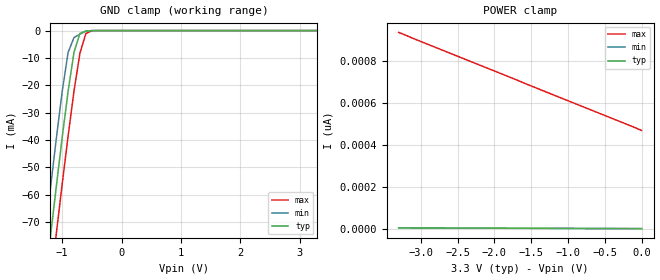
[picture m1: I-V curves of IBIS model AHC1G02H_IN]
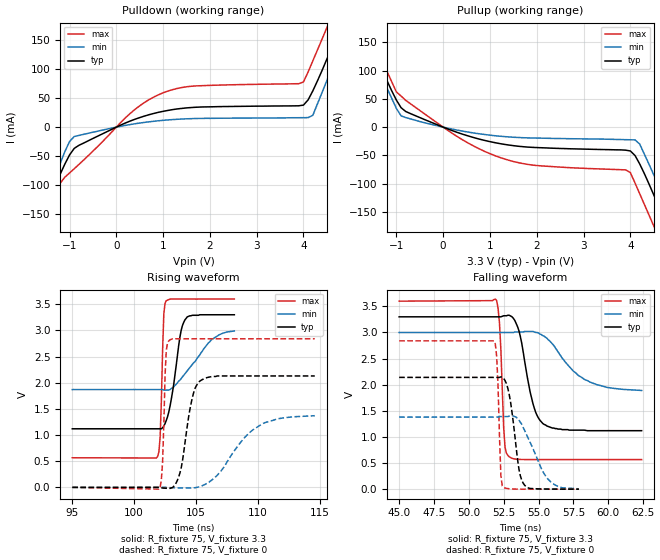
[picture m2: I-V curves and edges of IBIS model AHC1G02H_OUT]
| TEXAS INSTRUMENTS INCORPORATED
| Standard Linear and Logic Group
| IBIS Model of SN74AHC1G02H
| SINGLE 2-INPUT POSITIVE-NOR GATE
| CMPAK-5 5-pin (DCK) Package
[IBIS Ver]   2.1
[Comment Char]  |_char
[File name]   ul02_3c.ibs
[File Rev]   2.0
[Date]   May 11, 2000
[Source]   Data created from SPICE simulations at Hitachi,Ltd.
[Notes]   The following is an IBIS List for the AHC1G02H.
|   Please contact sllibis@ti.com with questions and
|   comments concerning SLL IBIS models.
[Disclaimer] Property of Texas Instruments Incorporated.  Unauthorized
   reproduction and/or distribution is strictly prohibited.
   This product is protected under copyright law.
   Created 2000, (C) Copyright 2000, Texas Instruments Inc.,
   All Rights Reserved.
   UNLESS THERE IS A SIGNED, WRITTEN AGREEMENT TO THE
   CONTRARY, TEXAS INSTRUMENTS () IS PROVIDING THE IBIS
   MODELS  AND WITHOUT ANY WARRANTY, EXPRESSED OR
   IMPLIED.  TI assumes no liability for:
   1) the accuracy of the IBIS models provided to your
   company;
   2) the proper functioning of these IBIS Models in your
   design or for any resulting applications; or
   3) infringement of patents, copyrights or intellectual
   property rights resulting from your use of these IBIS
   models.
   TI provides IBIS Models as a service to our customers.
   You and your company shall not distribute, sell or give
   these models to anyone else without prior written
   permission from TI.
   TI reserves the right to make changes to our products or
   to discontinue any semiconductor product or service
   without notice, and advises our customers to obtain the
   latest version of relevant information to verify, before
   placing orders, that the information being relied on is
   current.
   Please be aware that your receipt and use of the IBIS
   information provided shall serve as acceptance of these
   terms and conditions.  If you do not accept these terms,
   you should return or destroy the IBIS models and any
   other accompanying information immediately.
|   Component AHC1G02H
[Component]   AHC1G02H
[Manufacturer]   Hitachi, Ltd.
[Package]
|   typ   min   max
R_pkg   0.090   0.051   0.105
L_pkg   1.500nH   0.940nH   1.700nH
C_pkg   0.170pF   0.110pF   0.360pF
[Pin]   signal_name   model_name   R_pin   L_pin   C_pin
1   A   AHC1G02H_IN   0.098   1.590nH   0.110pF
2   B   AHC1G02H_IN   0.051   0.940nH   0.170pF
3   GND   GND   0.092   1.590nH   0.360pF
4   Y   AHC1G02H_OUT   0.105   1.700nH   0.110pF
5   VCC   POWER   0.104   1.690nH   0.110pF
| Models and submodels in the file (2): AHC1G02H_IN (Input), AHC1G02H_OUT (Output)
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|   Model AHC1G02H_IN
[Model]   AHC1G02H_IN
Model_type  Input
Polarity   Inverting
Vinl = 0.99
Vinh = 2.31
| variable   typ   min   max
C_comp   1.80pF   1.73pF   1.97pF
[Temperature Range]   25   85   -40
[Voltage Range]   3.3   3.0   3.6
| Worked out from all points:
|   GND clamp passes 1 mA (typ) near -0.70 V on its own axis
[GND Clamp]
|   Voltage   I(typ)   I(min)   I(max)
-3.3V     -486mA     -469mA     -503mA
-1.3V     -94.6mA    -76.9mA    -112mA
-1.2V     -75.8mA    -58.1mA    -93.1mA
-1.1V     -57.3mA    -39.8mA    -74.5mA
-1V       -39.2mA    -22.4mA    -56.2mA
-900mV    -22.2mA    -7.98mA    -38.6mA
-800mV    -7.87mA    -2.53mA    -22mA
-700mV    -1.03mA    -1.34mA    -8.2mA
-600mV    -206uA     -154uA     -1.06mA
-500mV    -11.2uA    -2.6uA     -57.2uA
3.3V      3.55pA     3.3pA      469pA
[POWER Clamp]
|   Voltage   I(typ)   I(min)   I(max)
-3.3V     7pA        6.6pA      934pA
-1.6V     5.23pA     4.9pA      694pA
-100mV    3.66pA     3.4pA      484pA
0V        3.55pA     3.3pA      469pA
|   Model AHC1G02H_OUT
[Model]   AHC1G02H_OUT
Model_type  Output
Polarity   Non-Inverting
Vmeas = 1.65
Cref = 15pf
| variable   typ   min   max
C_comp   3.84pF   3.72pF   3.96pF
[Temperature Range]   25   85   -40
[Voltage Range]   3.3   3.0   3.6
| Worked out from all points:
|   slope of the pulldown table from 0 to 0.495 V, typ, clamps not added: 30.4 ohm
|   slope of the pullup table from 0 to 0.495 V, typ, clamps not added: 34 ohm
|   rising waveform, R_fixture 75, V_fixture 3.3: 20-80 % time 792ps typ, 2.18ns min, 222ps max; typ from 1.12 V to 3.3 V
|   falling waveform, R_fixture 75, V_fixture 3.3: 20-80 % time 950ps typ, 2.23ns min, 265ps max; typ from 3.3 V to 1.12 V
|   falling waveform, R_fixture 75, V_fixture 0: 20-80 % time 607ps typ, 1.4ns min, 214ps max; typ from 2.14 V to 0 V
|   rising waveform, R_fixture 75, V_fixture 0: 20-80 % time 849ps typ, 2.7ns min, 216ps max; typ from 0 V to 2.13 V
[Pulldown]
|   Voltage   I(typ)   I(min)   I(max)
-3.3V     -489mA     -473mA     -506mA
-1.8V     -194mA     -179mA     -211mA
-1.6V     -156mA     -142mA     -173mA
-1.2V     -81mA      -62.6mA    -96.6mA
-900mV    -36.6mA    -16.1mA    -71.6mA
1V        27.2mA     11.7mA     59.1mA
3.9V      36.7mA     16.2mA     74.7mA
4.1V      47mA       16.4mA     95.1mA
4.5V      117mA      80.2mA     171mA
4.8V      174mA      137mA      229mA
5V        213mA      175mA      268mA
6.6V      528mA      491mA      584mA
[Pullup]
|   Voltage   I(typ)   I(min)   I(max)
-3.3V     491mA      474mA      508mA
-1.8V     196mA      179mA      214mA
-1.6V     157mA      141mA      175mA
-1V       47.9mA     33.1mA     62.4mA
-900mV    34.5mA     20mA       55.1mA
1.2V      -29mA      -16mA      -53.4mA
3.9V      -40.8mA    -22.2mA    -75.7mA
4.2V      -65.2mA    -30mA      -118mA
4.5V      -120mA     -84.4mA    -175mA
4.8V      -177mA     -138mA     -233mA
5V        -216mA     -177mA     -272mA
6.6V      -533mA     -494mA     -589mA
[Ramp]
| variable   typ   min   max
dV/dt_r   1.28E+00/8.40E-10   8.27E-01/2.73E-09   1.71E+00/2.10E-10
dV/dt_f   1.31E+00/9.40E-10   6.76E-01/2.31E-09   1.82E+00/2.60E-10
R_load = 75
[Rising Waveform]
R_fixture = 75
V_fixture = 3.3
V_fixture_min = 3.0
V_fixture_max = 3.6
|   Time   V(typ)   V(min)   V(max)
95ns      1.12V      1.87V      566mV
101.8ns   1.12V      1.87V      562mV
102.1ns   1.12V      1.87V      954mV
102.4ns   1.17V      1.86V      3.32V
102.6ns   1.28V      1.86V      3.57V
103.1ns   1.82V      1.9V       3.6V
103.8ns   3V         2.08V      3.6V
104.1ns   3.2V       2.17V      3.6V
106.2ns   3.3V       2.81V      3.6V
108.1ns   3.3V       2.99V      3.6V
[Falling Waveform]
R_fixture = 75
V_fixture = 3.3
V_fixture_min = 3.0
V_fixture_max = 3.6
|   Time   V(typ)   V(min)   V(max)
45ns      3.3V       3V         3.6V
52ns      3.3V       3V         3.61V
52.2ns    3.3V       3V         3.18V
52.6ns    3.32V      3V         800mV
52.9ns    3.33V      3V         620mV
53.6ns    3.03V      3.01V      570mV
54.6ns    1.64V      3.02V      566mV
55.3ns    1.26V      2.94V      566mV
58.3ns    1.13V      2.1V       566mV
62.4ns    1.12V      1.89V      566mV
[Falling Waveform]
R_fixture = 75
V_fixture = 0
|   Time   V(typ)   V(min)   V(max)
45ns      2.14V      1.38V      2.84V
51.8ns    2.14V      1.38V      2.84V
52ns      2.14V      1.38V      2.54V
52.3ns    2.15V      1.39V      261mV
52.4ns    2.14V      1.39V      61.8mV
52.9ns    1.81V      1.4V       7.58mV
53.6ns    378mV      1.32V      564uV
53.9ns    115mV      1.18V      175uV
55.7ns    2.3mV      187mV      -6uV
57.9ns    117uV      6.08mV     -3uV
[Rising Waveform]
R_fixture = 75
V_fixture = 0
|   Time   V(typ)   V(min)   V(max)
95ns      0V         0V         0V
102ns     -346uV     331uV      -34.1mV
102.3ns   -12.2mV    749uV      484mV
102.6ns   -17mV      -659uV     2.62V
102.9ns   -19.2mV    -5.28mV    2.82V
103.7ns   274mV      -9.53mV    2.84V
104.7ns   1.71V      -10.5mV    2.84V
105.3ns   2.03V      14.6mV     2.84V
110.4ns   2.13V      1.22V      2.84V
114.6ns   2.13V      1.37V      2.84V
